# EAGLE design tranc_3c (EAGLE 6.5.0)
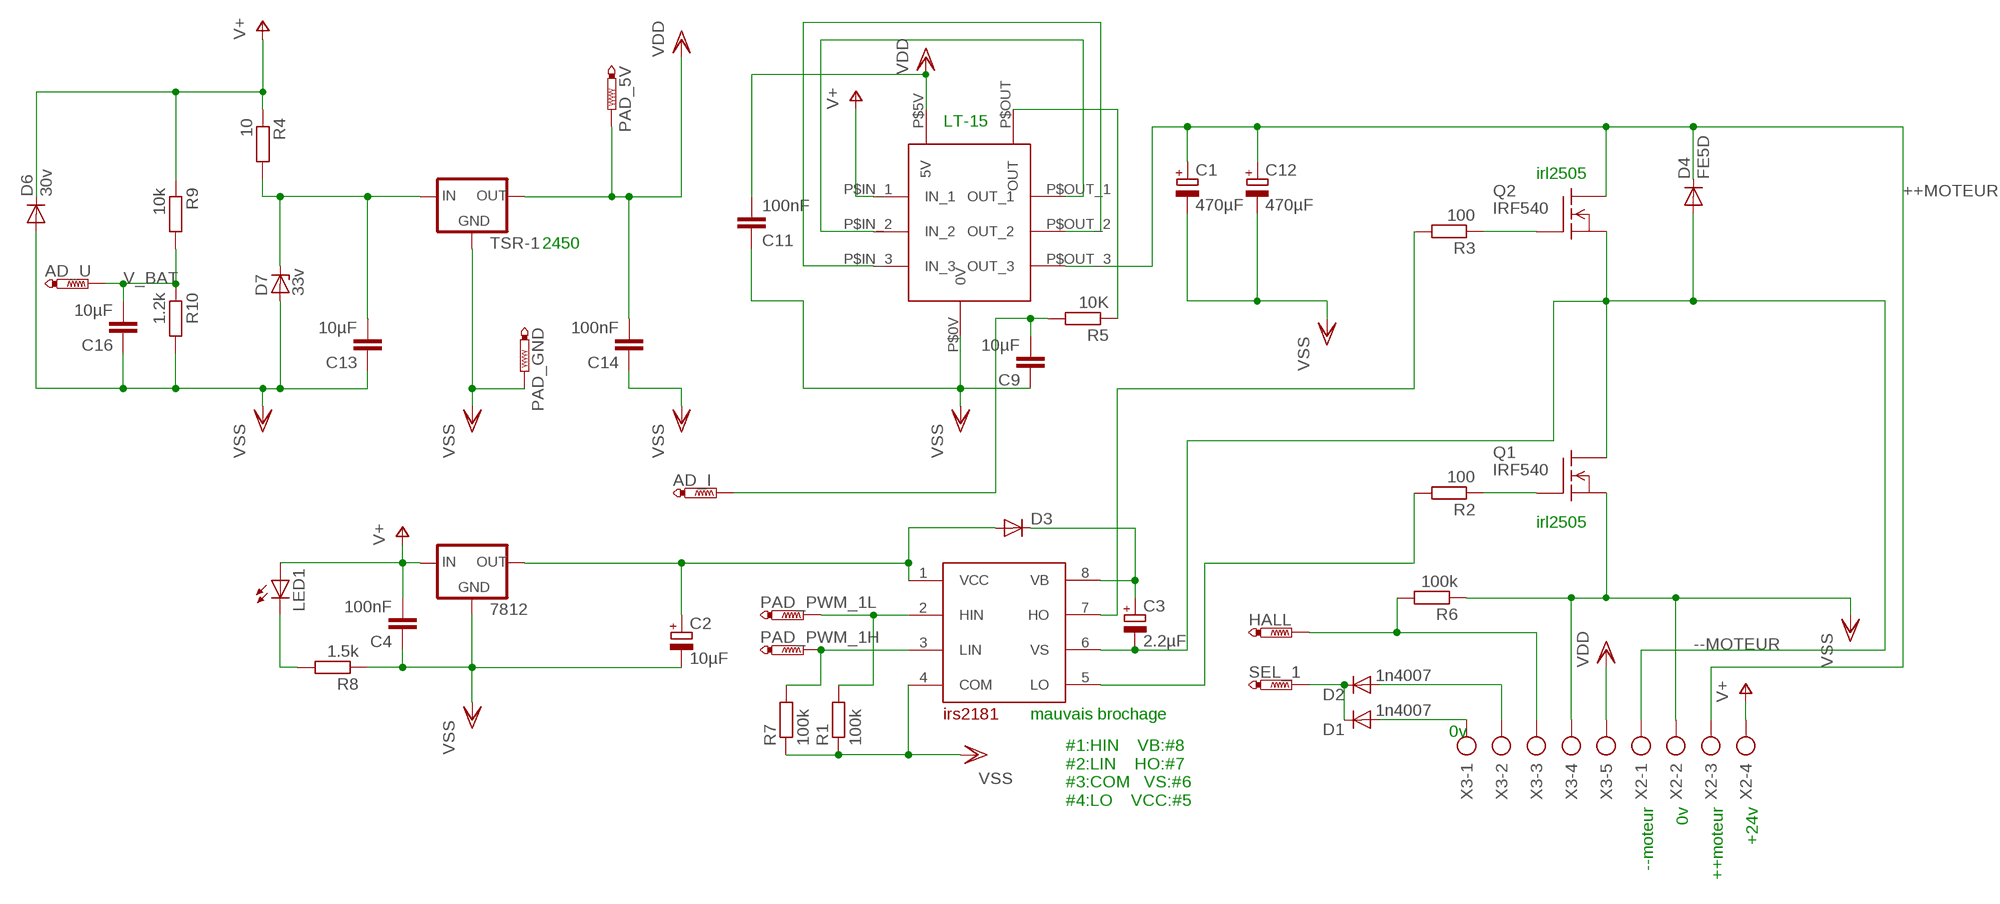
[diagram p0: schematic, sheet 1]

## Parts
7812  78XXS  [78XXS]
AD_I  PTR1TP20SQ  [TP20SQ]
AD_U  PTR1TP20SQ  [TP20SQ]
C1  470µF  CPOL-EUTT5D11L  [TT5D11L]
C2  10µF  CPOL-EUSMCB  [SMC_B]
C3  2.2µF  CPOL-EUSMCB  [SMC_B]
C4  100nF  C-EUC0805K  [C0805K]
C9  10µF  C-EUC1808  [C1808]
C11  100nF  C-EUC0805K  [C0805K]
C12  470µF  CPOL-EUTT5D11L  [TT5D11L]
C13  10µF  C-EUC1808  [C1808]
C14  100nF  C-EUC0805K  [C0805K]
C16  10µF  C-EUC1808  [C1808]
D1  1n4007  DIODE-MINIMELF  [MINIMELF]
D2  1n4007  DIODE-MINIMELF  [MINIMELF]
D3  DIODE-MINIMELF  [MINIMELF]
D4  FE5D  [G4-12]
D6  30v  BY550  [DO27-15]
D7  33v  ZENER-DIODESOD80C  [SOD80C]
HALL  PTR1TP20SQ  [TP20SQ]
LED1  LEDB152  [Q62902-B152]
PAD_5V  PTR1TP20SQ  [TP20SQ]
PAD_GND  PTR1TP20SQ  [TP20SQ]
PAD_PWM_1H  PTR1TP20SQ  [TP20SQ]
PAD_PWM_1L  PTR1TP20SQ  [TP20SQ]
Q1  IRF540  [TO220]
Q2  IRF540  [TO220]
R1  100k  R-EU_M1206  [M1206]
R2  100  R-EU_M0805  [M0805]
R3  100  R-EU_M0805  [M0805]
R4  10  R-EU_M1206  [M1206]
R5  10K  R-EU_M0805  [M0805]
R6  100k  R-EU_M0805  [M0805]
R7  100k  R-EU_M0805  [M0805]
R8  1.5k  R-EU_0309/10  [0309/10]
R9  10k  R-EU_M0805  [M0805]
R10  1.2k  R-EU_M0805  [M0805]
SEL_1  PTR1TP20SQ  [TP20SQ]
TSR-1  78XXS  [78XXS]
U$1  LTS25-NP  [LTS25]
U$2  IRS2181  [SO08]
X2  AK300/4  [AK300/4]
X3  AK300/5  [AK300/5]

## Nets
++MOTEUR: C1.+ C12.+ D4.C Q2.2(D) U$1.P$OUT_3(OUT_3) X2.3
--MOTEUR: C3.- D4.A Q1.2(D) Q2.3(S) U$2.6(VS) X2.1
N$1: Q1.1(G) R2.1
N$2: U$1.P$IN_2(IN_2) U$1.P$OUT_1(OUT_1)
N$3: HALL.TP R6.2 X3.3
N$4: D2.A X3.2
N$5: U$1.P$IN_3(IN_3) U$1.P$OUT_2(OUT_2)
N$6: D1.C D2.C SEL_1.TP
N$8: R5.1 U$1.P$OUT(OUT)
N$10: Q2.1(G) R3.1
N$11: R2.2 U$2.5(LO)
N$12: D1.A X3.1
N$13: C13.2 D7.C R4.2 TSR-1.IN
N$14: C3.+ D3.C U$2.8(VB)
N$15: 7812.OUT C2.+ D3.A U$2.1(VCC)
N$16: PAD_PWM_1L.TP R1.2 U$2.2(HIN)
N$17: PAD_PWM_1H.TP R7.2 U$2.3(LIN)
N$18: R3.2 U$2.7(HO)
N$19: LED1.K(C) R8.2
N$30: AD_I.TP C9.2 R5.2
V+: 7812.IN C4.2 D6.C LED1.A R4.1 R9.1 U$1.P$IN_1(IN_1) X2.4
V_BAT: AD_U.TP C16.2 R9.2 R10.1
VDD: C11.2 C14.2 PAD_5V.TP TSR-1.OUT U$1.P$5V(5V) X3.5
VSS: 7812.GND C1.- C2.- C4.1 C9.1 C11.1 C12.- C13.1 C14.1 C16.1 D6.A D7.A PAD_GND.TP Q1.3(S) R1.1 R6.1 R7.1 R8.1 R10.2 TSR-1.GND U$1.P$0V(0V) U$2.4(COM) X2.2 X3.4

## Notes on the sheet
- LT-15
- irl2505
- 2450
- irl2505
- mauvais brochage
- 0v
- --moteur | 0v | ++moteur | +24v
- #1:HIN    VB:#8
  #2:LIN    HO:#7
  #3:COM   VS:#6
  #4:LO    VCC:#5

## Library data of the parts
7812 TSR-1 = v-reg:78XXS: VOLTAGE REGULATOR
AD_I AD_U HALL PAD_5V PAD_GND PAD_PWM_1H PAD_PWM_1L SEL_1 = testpad:PTR1: TEST PIN
C1-C3 C12 = rcl:CPOL-EU: POLARIZED CAPACITOR, European symbol
C4 C9 C11 C13 C14 C16 = rcl:C-EU: CAPACITOR, European symbol
D1-D3 = diode:DIODE-: DIODE
D4 = diode:FE5D: DIODE
D6 = diode:BY550: DIODE
D7 = diode:ZENER-DIODE: Z-Diode
LED1 = led:LED: LED
Q1 Q2 = transistor-fet:IRF540: N-Channel Enhancement MOSFET (HEXFET); 100V; 28A; 0,077Ohm
R1-R10 = rcl:R-EU_: RESISTOR, European symbol
U$1 = lem:LTS25-NP
U$2 = ir:IRS2181
X2 = con-ptr500:AK300/4: CONNECTOR; OC_FARNELL: unknown; OC_NEWARK: unknown
X3 = con-ptr500:AK300/5: CONNECTOR; OC_FARNELL: unknown; OC_NEWARK: unknown

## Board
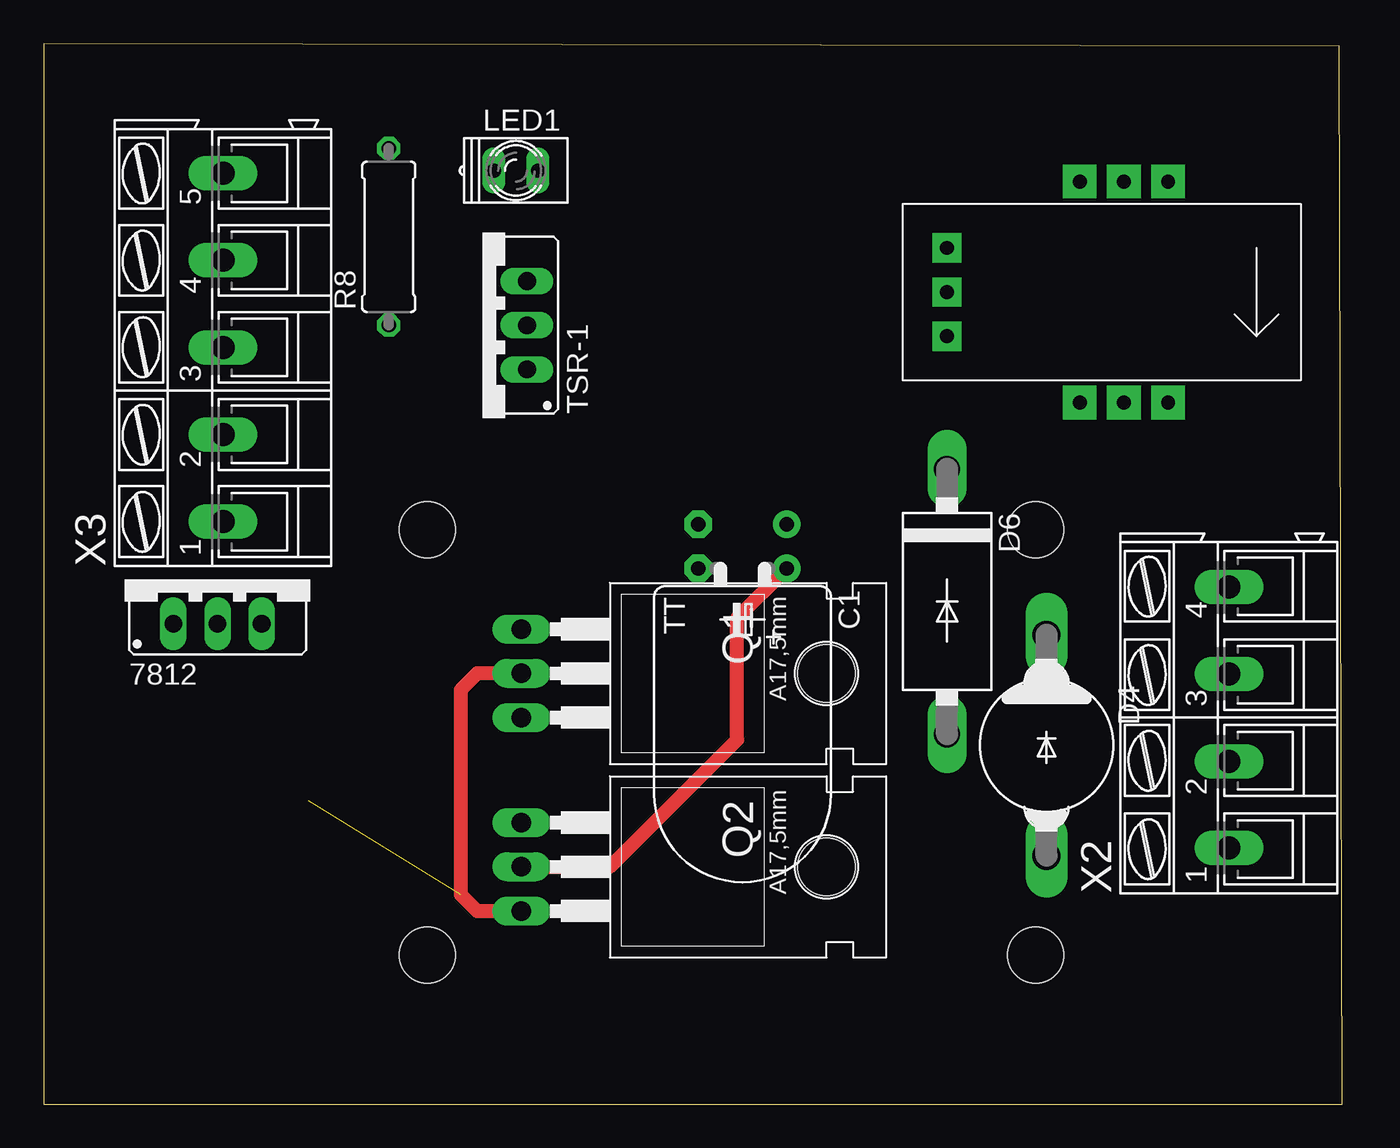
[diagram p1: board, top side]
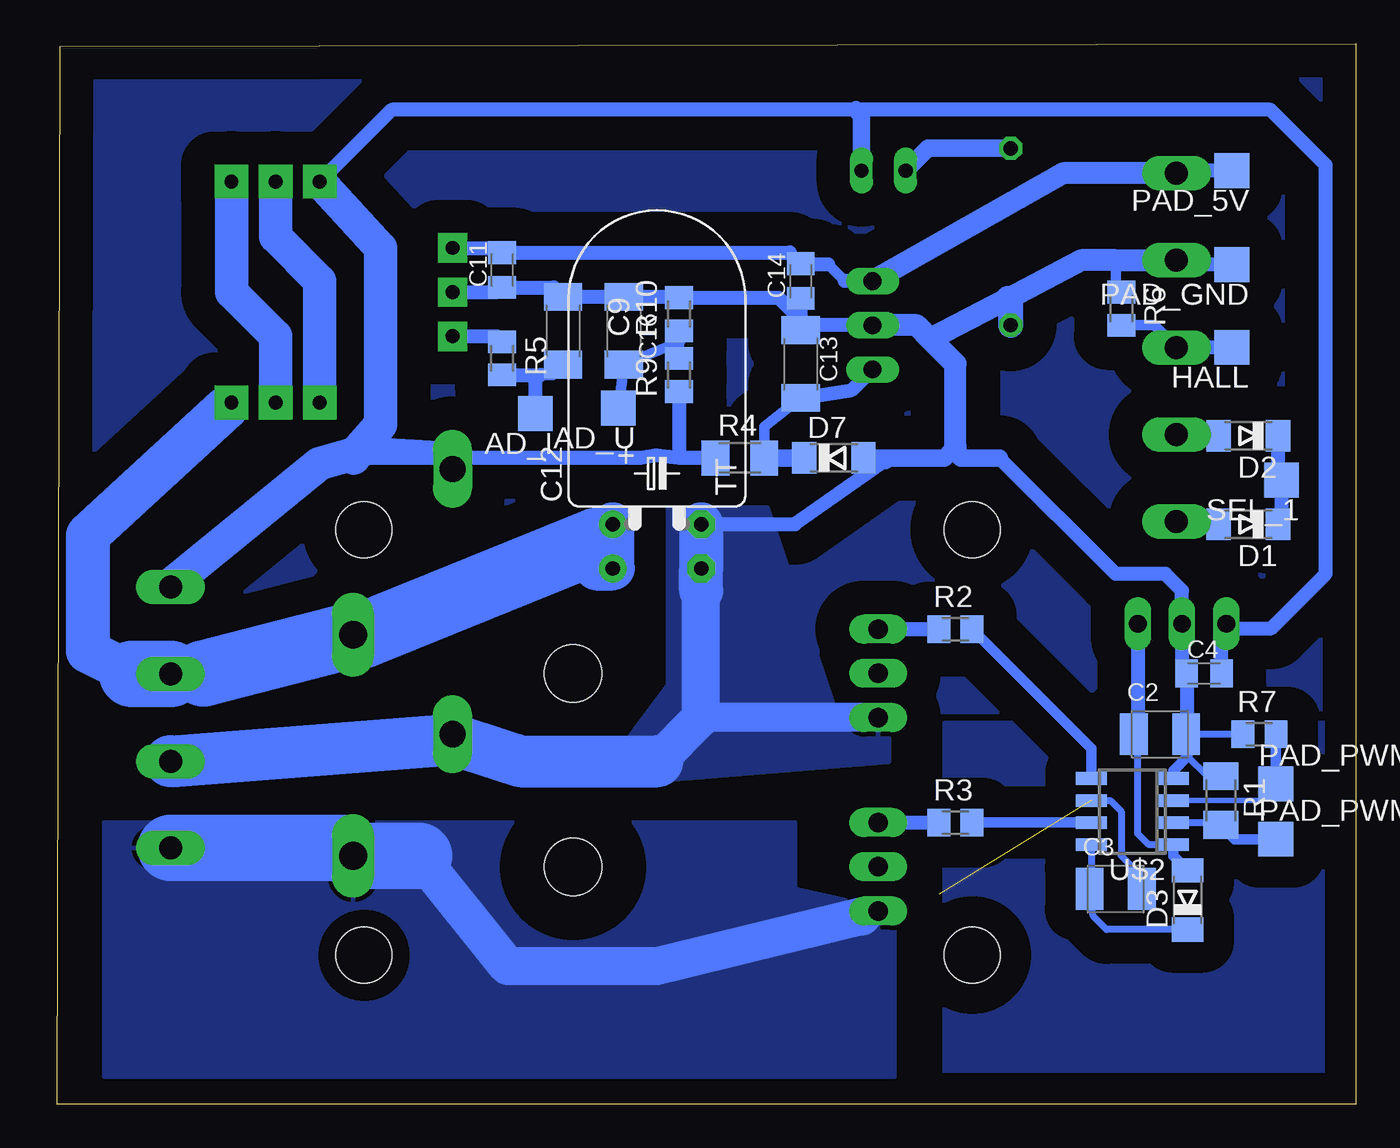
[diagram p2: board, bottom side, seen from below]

Size 74.6 x 60.95 mm. Coordinates in mm from the lower left corner, seen from the top.
Outline: 0,0 74.6,0 74.45,60.79 0,60.95 0,0
Copper layers (1*16): Top 0.035mm / dielectric 1.5mm / Bottom 0.035mm
Design rules "default": minimum track width 10mil, minimum drill 24mil, track to track 8mil, track to pad 8mil, pad to pad 8mil, via to via 8mil, smd to smd 8mil, copper to edge 40mil, drill to drill 8mil, minimum pad ring 10mil, minimum via ring 8mil, stop-mask expansion 4mil, vias tented up to drill 0mil, thermal gap 10mil
Holes 3.2 mm at 56.98,8.57 22.06,8.57 22.06,33.02 56.98,33.02

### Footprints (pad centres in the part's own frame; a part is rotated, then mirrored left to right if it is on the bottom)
78XXS = drill 1.016 long: GND 0,-2.54; IN -2.54,-2.54; OUT 2.54,-2.54
TP20SQ = smd 2 x 2: TP 0,0
TT5D11L = drill 0.813 pad 1.6: + -2.54,0 | drill 0.813 pad 1.6 octagon: - 2.54,0
SMC_B = smd 1.6 x 2.4: + -1.5,0; - 1.5,0
C0805K = smd 1.3 x 1.6: 1 -1,0; 2 1,0
C1808 = smd 1.6 x 2.2: 1 -1.95,0; 2 1.95,0
MINIMELF = smd 1.4 x 1.8: A 1.7,0; C -1.7,0
G4-12 = drill 1.6 long: A 6.35,0; C -6.35,0
DO27-15 = drill 1.499 long: A 7.62,0; C -7.62,0
SOD80C = smd 1.4 x 1.8: A 1.7,0; C -1.7,0
Q62902-B152 = drill 0.813 long: A 1.27,0; K -1.27,0
TO220 = drill 1.118 long: 1 -2.54,-6.35; 2 0,-6.35; 3 2.54,-6.35 | hole 3.302: 0,11.176
M1206 = smd 1.6 x 2: 1 -1.4,0; 2 1.4,0
M0805 = smd 1.3 x 1.6: 1 -0.95,0; 2 0.95,0
0309/10 = drill 0.813 octagon: 1 -5.08,0; 2 5.08,0
LTS25 = drill 0.8 pad 1.676 square: P$0V -10.16,0; P$5V -10.16,2.54; P$OUT -10.16,-2.54 | drill 0.8 pad 1.93 square: P$IN_1 -2.54,6.35; P$IN_2 0,6.35; P$IN_3 2.54,6.35; P$OUT_1 -2.54,-6.35; P$OUT_2 0,-6.35; P$OUT_3 2.54,-6.35
SO08 = smd 0.72 x 1.78: 1 -1.905,-2.35; 2 -0.635,-2.35; 3 0.635,-2.35; 4 1.905,-2.35; 5 1.905,2.35; 6 0.635,2.35; 7 -0.635,2.35; 8 -1.905,2.35
AK300/4 = drill 1.321 long: 1 -7.493,0; 2 -2.515,0; 3 2.515,0; 4 7.493,0
AK300/5 = drill 1.321 long: 1 -10.008,0; 2 -5.004,0; 3 0,0; 4 5.004,0; 5 10.008,0

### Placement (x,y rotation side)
7812  10,30.16 0 top
AD_I  47.14,39.68 180 bottom
AD_U  42.38,40 180 bottom
C1  40.16,30.79 180 top
C2  11.27,21.27 0 bottom
C3  13.81,12.38 0 bottom
C4  8.73,24.76 0 bottom
C9  45.55,44.45 270 bottom
C11  49.05,47.94 90 bottom
C12  40.16,33.33 0 bottom
C13  31.9,42.54 270 bottom
C14  31.9,47.3 90 bottom
C16  42.06,44.45 270 bottom
D1  6.18,33.33 180 bottom
D2  6.18,38.41 180 bottom
D3  9.68,11.74 90 bottom
D4  57.62,20.63 270 top
D6  51.91,28.89 270 top
D7  30,37.14 0 bottom
HALL  7.14,43.49 180 bottom
LED1  27.14,53.65 0 top
PAD_5V  7.14,53.65 180 bottom
PAD_GND  7.14,48.26 180 bottom
PAD_PWM_1H  4.6,18.41 0 bottom
PAD_PWM_1L  4.6,15.24 0 bottom
Q1  33.81,24.76 270 top
Q2  33.81,13.65 270 top
R1  7.77,17.46 270 bottom
R2  23.01,27.3 0 bottom
R3  23.01,16.19 0 bottom
R4  35.39,37.14 0 bottom
R5  49.05,42.86 270 bottom
R6  13.49,45.72 270 bottom
R7  5.55,21.27 0 bottom
R8  19.84,49.84 90 top
R9  38.89,41.91 90 bottom
R10  38.89,45.4 90 bottom
SEL_1  4.28,35.87 180 bottom
TSR-1  25.23,44.76 90 top
U$1  62.06,46.67 0 top
U$2  12.85,16.82 90 bottom
X2  68.1,22.22 90 top
X3  10.31,43.49 90 top

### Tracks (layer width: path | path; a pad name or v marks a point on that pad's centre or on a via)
++MOTEUR
  Top 0.813: Q2.2 32.54,13.65 39.84,20.95 39.84,27.93 C1.+
  Bottom 1.27: U$1.P$OUT_3 64.92,40
  Bottom 2.184: D4.C 56.98,26.98
  Bottom 2.54: 70.3,24.73 72.86,26.03 72.86,32.7 64.92,40 | C12.+ C1.+ 43.65,30.79 43.65,32.38 | X2.3 67.46,24.76 66.19,24.76 65.56,24.76
  Bottom 3.81: X2.3 70.3,24.73 | 56.98,26.98 43.65,32.38 | 66.19,24.76 D4.C
--MOTEUR  (1 unrouted)
  Top 0.813: Q1.2 24.92,24.76 23.96,23.81 23.96,12.06 24.92,11.11 Q2.3
  Bottom 0.406: U$2.6 14.12,17.46 13.49,16.82 13.49,14.28 12.22,13.01 12.22,12.47 C3.-
  Bottom 1.676: Q2.3 28.41,10.79 | 58.06,14.73 D4.A
  Bottom 2.184: 28.41,10.79 40.16,7.93 48.73,7.93 53.81,14.28
  Bottom 3.81: X2.1 58.06,14.73 | 53.81,14.28 D4.A
  pour Bottom: 26.5,11.11 26.5,1.58 71.91,1.58 71.91,16.19 32.22,16.19 32.22,12.38
N$1
  Bottom 0.813: Q1.1 R2.1
N$2
  Bottom 1.93: U$1.P$IN_2 62.06,49.84 59.52,47.3 U$1.P$OUT_1
N$3
  Bottom 0.61: R6.2 11.59,44.77 X3.3
  Bottom 0.813: HALL.TP X3.3
N$4
  Bottom 0.61: 10.24,38.41 X3.2
  Bottom 0.813: D2.A 10.24,38.41
N$5
  Bottom 1.93: U$1.P$IN_3 64.61,46.67 62.06,44.13 U$1.P$OUT_2
N$6
  Bottom 0.61: 4.48,36.08 SEL_1.TP | 4.28,33.54 D1.C
  Bottom 0.813: D2.C 4.48,36.08 | SEL_1.TP 4.28,33.54
N$8
  Bottom 0.61: 49.37,44.13 R5.1
  Bottom 0.813: U$1.P$OUT 49.37,44.13
N$9
  pour Bottom (isolate 1.93): 0.15,60.64 74.13,60.64 74.45,22.54 0.47,22.54
N$10
  Bottom 0.813: Q2.1 R3.1
N$11
  Bottom 0.61: U$2.5 15.2,20.44 R2.2
N$12
  Bottom 0.61: 10.16,33.33 X3.1
  Bottom 0.813: D1.A 10.16,33.33
N$13
  Bottom 0.61: R4.2 33.99,38.95 C13.2
  Bottom 0.813: C13.2 28.96,41.04 TSR-1.IN
  Bottom 1.016: R4.2 D7.C
N$14
  Bottom 0.406: U$2.8 15.2,12.48 C3.+ 15.39,12.29 15.08,10.79 14.33,10.04 D3.C
N$15
  Bottom 0.406: U$2.1 11.9,14.92 12.54,15.55 12.54,21.18
  Bottom 0.61: 12.54,21.18 C2.+ | U$2.1 10.5,14.27 D3.A
  Bottom 0.813: 7812.OUT 12.54,21.5 C2.+
N$16
  Bottom 0.406: U$2.2 7.9,16.19 R1.2
  Bottom 0.61: PAD_PWM_1L.TP 6.95,15.24 R1.2
N$17
  Bottom 0.305: U$2.3 5.55,17.46 PAD_PWM_1H.TP
  Bottom 0.406: PAD_PWM_1H.TP
  Bottom 0.61: R7.2 PAD_PWM_1H.TP
N$18
  Bottom 0.61: U$2.7 R3.2
N$19
  Bottom 1.016: R8.2 24.6,54.92 LED1.K
N$20
  pour Bottom (isolate 1.778): 0.79,21.9 0.79,1.27 23.65,1.27 23.65,21.9 1.1,21.9
N$30
  Bottom 0.61: C9.2 46.14,41.91 46.82,41.91 47.14,41.59
  Bottom 0.813: R5.2 46.82,41.91 | AD_I.TP 47.14,41.59
V+
  Bottom 0.406: 57.63,37.78 57.31,37.57
  Bottom 0.61: 39.12,41.04 R9.1 | 38.89,37.14 39.75,37.14 40.21,37.29
  Bottom 0.813: R9.1 38.89,37.14 | 38.89,37.14 40.21,37.29 41.11,37.14 57.59,37.14 | R4.1 38.89,37.14 | C4.2 7.72,27.35 | 7.72,27.35 7812.IN | 7.72,27.35 4.87,27.35 1.74,30.47 1.74,53.97 4.92,57.15 28.73,57.15 55.4,57.15 U$1.P$IN_1
  Bottom 1.016: LED1.A 28.41,56.83 28.73,57.15
  Bottom 1.27: 57.3,37.46 57.21,37.71 | X2.4 68.1,29.84 | D6.C 52.22,36.51 52.22,37.46 57.63,37.78
  Bottom 1.93: 57.3,37.46 59.52,36.83 68.1,29.84 | U$1.P$IN_1 56.03,49.21 56.03,39.05 57.21,37.71 57.31,37.57 57.59,37.14
V_BAT
  Bottom 0.61: R9.2 R10.1 38.84,43.81 C16.2 AD_U.TP
VDD
  Bottom 0.61: 49.32,49.21 C11.2 | 29.36,47.3 30.31,48.26 | 31.86,48.26 C14.2 32.54,48.94 | 10.16,53.65 X3.5
  Bottom 0.813: U$1.P$5V 49.32,49.21 | TSR-1.OUT 29.36,47.3 | 30.31,48.26 31.86,48.26 | C11.2 32.54,48.94 | PAD_5V.TP 10.16,53.65
  Bottom 1.27: X3.5 16.81,53.5 TSR-1.OUT
VSS
  Bottom 0.406: R1.1 8.54,18.86 9.68,20 | R7.1 C2.-
  Bottom 0.61: 49.32,46.67 C11.1 | 46.1,46.94 C9.1 | 31.58,44.76 31.9,44.76 | 41.75,46.4 C16.1 | 39.25,46.4 R10.2 | 13.81,46.66 13.81,48.5 | U$2.4 10.5,19.17 9.68,20 9.68,21.18 C2.-
  Bottom 0.813: U$1.P$0V 49.32,46.67 | C11.1 46.1,46.94 | TSR-1.GND 31.58,44.76 33.17,46.35 R10.2 | C13.1 31.9,44.76 C14.1 | C9.1 41.75,46.4 | C16.1 39.25,46.4 | PAD_GND.TP 10.07,48.26 X3.4 | C12.- 32.22,33.33 27.03,36.99 26.82,37.14 | C2.- 9.73,21.31 C4.1 10,25.03 7812.GND 10,29.52 10.95,30.47 13.81,30.47 20.47,37.14 | 13.81,46.66 R6.1
  Bottom 1.016: 23.17,37.62 23.65,37.14 D7.A 27.18,37.14 27.03,36.99 | 23.17,37.62 23.01,37.78 | 20.47,37.14 22.7,37.14 23.17,37.62
  Bottom 1.27: 23.01,37.78 23.01,42.54 24.44,43.97 | 24.44,43.97 25.23,44.76 TSR-1.GND | 24.44,43.97 19.98,46.3 15.79,48.5 13.81,48.5 X3.4 | D6.A 51.91,20.97
  Bottom 1.422: R8.1 19.84,46.16 19.98,46.3
  Bottom 1.676: Q1.3 37.62,22.22
  Bottom 2.184: 40.13,19.7 37.62,22.22 37.62,29.52
  Bottom 2.54: C12.- C1.- 37.62,29.52
  Bottom 3: X2.2 51.91,20.97 48,19.7 40.13,19.7
  pour Bottom: 30,22.86 33.81,34.29 39.52,34.29 39.52,24.12 42.38,20.31 42.38,18.41 26.82,19.68 26.82,22.54

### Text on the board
Bottom: trancannage bottom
